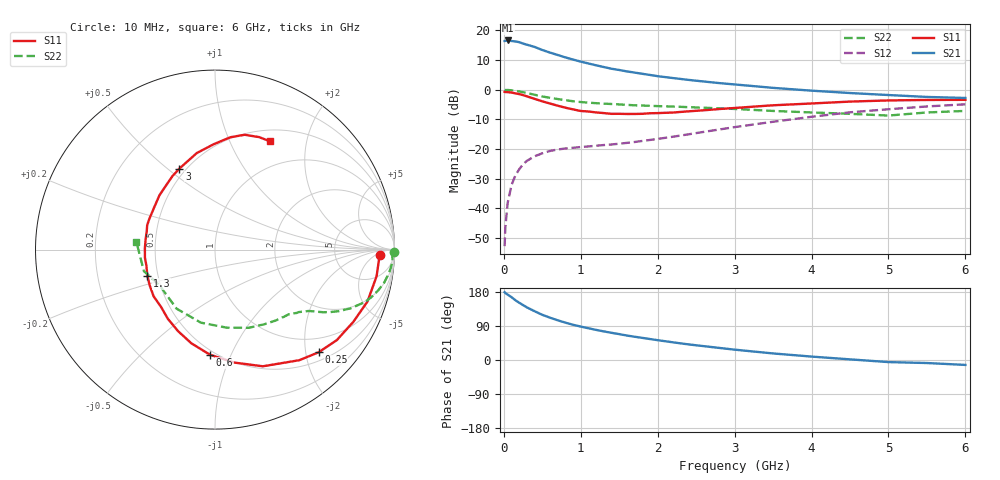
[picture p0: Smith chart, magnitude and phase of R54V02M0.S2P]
! SIEMENS Small Signal Semiconductors
! BFR183
! Si NPN RF Bipolar Junction Transistor in SOT23
! VCE = 4 V  IC = 2 mA
! Common Emitter S-Parameters:  May  1996
# GHz  S  MA  R  50
!  f  S11  S21  S12  S22
! GHz  MAG  ANG  MAG  ANG  MAG  ANG  MAG  ANG
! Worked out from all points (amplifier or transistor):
!   36 points, 10 MHz to 6 GHz, reference 50 ohm
!   highest |S21| = 16.6 dB at 50 MHz (marker M1)
!   |S21| within 3 dB of that: start of sweep to 478.5 MHz
!   unconditionally stable (mu >= 1): 1.389 GHz to 2.835 GHz
!   at 250 MHz: K = 0.23, MSG = 20.4 dB, |S12| = -25.1 dB
!   at 1.4 GHz: K = 1.01, MAG = 12.3 dB, |S12| = -18.5 dB
!   at 6 GHz: K = 0.91, MSG = 1.1 dB, |S12| = -4.9 dB
!   S11 on the Smith chart (normalised r, x): 10 MHz: 21, -8; 250 MHz: 0.67, -2.26; 600 MHz: 0.47, -0.84; 1.3 GHz: 0.44, -0.15; 3 GHz: 0.46, +0.55; 6 GHz: 0.64, +1.43
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0.01  0.921 -1.9  6.653 178.9  0.0023 91.8  0.9964 -0.8
0.02  0.9153 -3.6  6.669 176.9  0.0049 90.1  0.9871 -1.5
0.05  0.9124 -9.4  6.79 172.6  0.0124 84.5  0.9919 -3.8
0.1  0.8974 -18.8  6.651 165.7  0.0247 79.9  0.9796 -7.4
0.15  0.8695 -27.6  6.525 157.8  0.0359 73.8  0.9607 -11.0
0.2  0.8456 -36.6  6.352 151.1  0.0456 70.1  0.9368 -14.1
0.25  0.813 -44.7  6.017 144.9  0.0555 65.3  0.9101 -17.0
0.3  0.7747 -52.7  5.76 138.8  0.0633 62.1  0.8829 -19.4
0.4  0.7027 -67.7  5.28 128.7  0.0755 55.8  0.8236 -23.4
0.5  0.6379 -80.5  4.685 119.2  0.0848 51.1  0.7708 -26.4
0.6  0.5864 -92.7  4.236 111.7  0.0929 47.6  0.7316 -28.4
0.8  0.4987 -114.4  3.518 98.6  0.1024 43.5  0.6666 -31.3
0.9  0.4664 -124.3  3.233 92.9  0.1051 43.1  0.6405 -32.4
1.1  0.4296 -142.8  2.776 83.8  0.1108 42.8  0.6066 -34.7
1.3  0.4043 -158.8  2.416 75.5  0.1169 43.6  0.5834 -36.6
1.7  0.3909 171.4  1.95 61.4  0.1316 48.3  0.5465 -41.3
2.2  0.4131 144.8  1.576 46.6  0.1616 53.0  0.5215 -49.0
3  0.4931 113.7  1.23 27.3  0.2343 54.1  0.475 -66.5
3.5  0.5473 100.7  1.077 17.3  0.2887 50.7  0.4395 -81.6
4.5  0.6319 82.2  0.881 1.7  0.4166 39.1  0.3926 -123.0
5.5  0.6734 68.5  0.757 -8.0  0.5232 24.5  0.4141 -163.2
6  0.6766 63.0  0.727 -13.0  0.5685 15.3  0.4399 174.4
